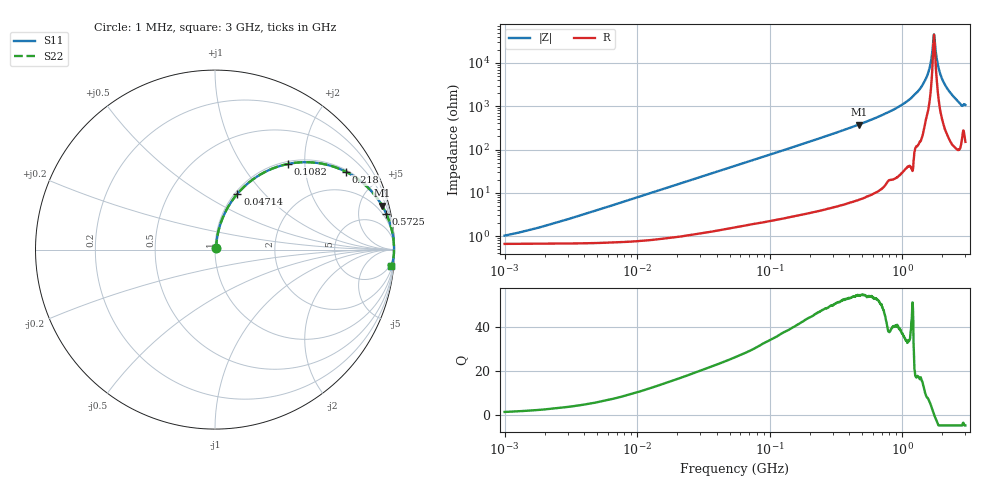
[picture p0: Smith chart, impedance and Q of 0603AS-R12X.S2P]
!s-Parameter Generated by FASTRON Sdn. Bhd.
!FASTRON P/N : 0603AS-R12X
!Keysight Technologies: E4991B_MY54100416_A.01.15
!Date created: Wed Oct 04 13:28:29 2023
!Version  : Rev01 Wed Oct 04 13:28:29 2023
!Data & Calibration Information:
!Freq	S11	S21	S12	S22
!PortZ  Port1:50+j0  Port2:50+j0
!When reading reference impedance value at option line is always used.
! Remarks : This data is being provided solely for informational purposes.
# Hz S dB R 50
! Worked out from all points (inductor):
!   1601 points, 1 MHz to 3 GHz, reference 50 ohm
!   read as one part in series: L = 125 nH near 2.562 MHz
!   highest Q = 54.8 at 471 MHz (marker M1), where L = 127 nH
!   self-resonance near 1.739 GHz
!   S11 on the Smith chart (normalised r, x): 1 MHz: 1.01, +0.02; 47.14 MHz: 1.03, +0.72; 108.2 MHz: 1.05, +1.64; 218 MHz: 1.07, +3.31; 572.5 MHz: 1.17, +9.50; 3 GHz: 4, -21
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1000000  -39.81 49.6  -0.06 -0.4  -0.06 -0.4  -39.81 49.6
3804036  -30.33 75.4  -0.06 -1.7  -0.06 -1.7  -30.33 75.4
1.447069e7  -19.06 79.3  -0.13 -6.4  -0.13 -6.4  -19.06 79.3
4.713729e7  -9.49 68.1  -0.64 -19.6  -0.64 -19.6  -9.49 68.1
5.477226e7  -8.38 65.4  -0.82 -22.4  -0.82 -22.4  -8.38 65.4
1.081723e8  -4.08 49.7  -2.35 -38.7  -2.35 -38.7  -4.08 49.7
2.083556e8  -1.54 31.9  -5.53 -56.8  -5.53 -56.8  -1.54 31.9
2.179536e8  -1.43 30.8  -5.82 -58.0  -5.82 -58.0  -1.43 30.8
4.710174e8  -0.33 14.8  -11.86 -74.2  -11.86 -74.2  -0.33 14.8
5.725215e8  -0.22 11.8  -13.75 -77.1  -13.75 -77.1  -0.22 11.8
7.925923e8  -0.11 7.7  -17.44 -80.8  -17.44 -80.8  -0.11 7.7
1.113852e9  -0.04 4.2  -22.75 -84.1  -22.75 -84.1  -0.04 4.2
1.381259e9  -0.03 2.1  -28.53 -84.5  -28.53 -84.5  -0.03 2.1
1.565327e9  -0.02 1.0  -35.11 -81.3  -35.11 -81.3  -0.02 1.0
1.629261e9  -0.02 0.6  -39.08 -78.2  -39.08 -78.2  -0.02 0.6
1.695807e9  -0.02 0.2  -46.36 -63.1  -46.36 -63.1  -0.02 0.2
1.738771e9  -0.02 0.0  -53.16 -2.1  -53.16 -2.1  -0.02 0.0
1.782824e9  -0.02 -0.2  -46.64 58.8  -46.64 58.8  -0.02 -0.2
1.921792e9  -0.02 -0.9  -35.67 80.3  -35.67 80.3  -0.02 -0.9
2.092429e9  -0.03 -1.8  -30.17 82.7  -30.17 82.7  -0.03 -1.8
2.727913e9  -0.10 -4.9  -21.36 79.9  -21.36 79.9  -0.10 -4.9
3e9  -0.15 -5.2  -20.75 76.7  -20.75 76.7  -0.15 -5.2
